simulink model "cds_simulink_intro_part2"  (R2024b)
settings: Solver=ode15s  StartTime=0.0  StopTime=30.0  RelTol=1e-3
undefined symbols (not defined in the file or in its folder): param

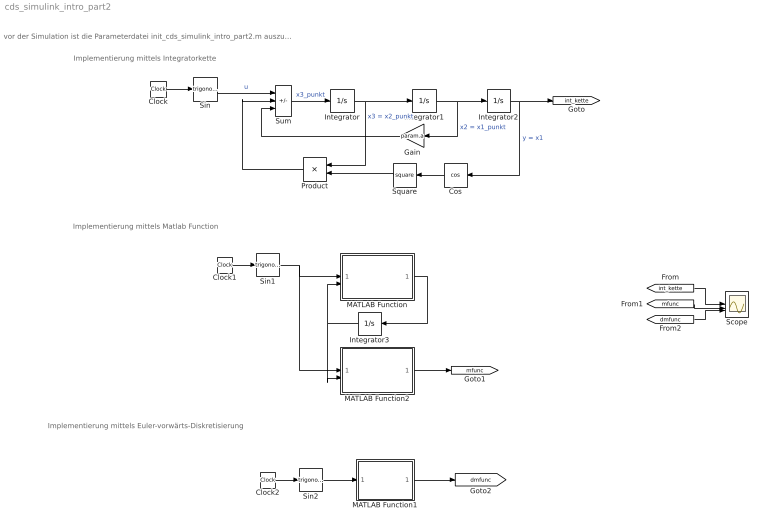
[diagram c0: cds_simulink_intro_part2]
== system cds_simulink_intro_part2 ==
  note: Implementierung mittels Matlab Function
  note: Implementierung mittels Integratorkette
  note: Implementierung mittels Euler-vorwärts-Diskretisierung
  note: vor der Simulation ist die Parameterdatei init_cds_simulink_intro_part2.m auszuführen
  Clock : Clock
  Clock1 : Clock
  Clock2 : Clock
  Cos : Trigonometry  Operator=cos
  Gain : Gain  Gain=param.a
  Integrator : Integrator
  Integrator1 : Integrator
  Integrator2 : Integrator
  Integrator3 : Integrator  InitialCondition=[0;0;0]
  MATLAB Function : MATLAB Function  TreatAsAtomicUnit=on
  MATLAB Function1 : MATLAB Function  TreatAsAtomicUnit=on
  MATLAB Function2 : MATLAB Function  TreatAsAtomicUnit=on
  Product : Product
  Scope : Scope  NumInputPorts=3
  Sin : Trigonometry
  Sin1 : Trigonometry
  Sin2 : Trigonometry
  Square : Math  Operator=square
  Sum : Sum  Inputs=---
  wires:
  Sin/1 -> Sum/1  "u"
  Integrator/1 -> Product/1, Integrator1/1  "x3 = x2_punkt"
  Sum/1 -> Integrator/1  "x3_punkt"
  Integrator1/1 -> Gain/1, Integrator2/1  "x2 = x1_punkt"
  Integrator2/1 -> [int_kette], Cos/1  "y = x1"
  Cos/1 -> Square/1
  Square/1 -> Product/2
  Product/1 -> Sum/2
  Clock/1 -> Sin/1
  Sin1/1 -> MATLAB Function2/1(u), MATLAB Function/1(u)
  Integrator3/1 -> MATLAB Function2/2(xx), MATLAB Function/2(xx)
  Clock1/1 -> Sin1/1
  Gain/1 -> Sum/3
  Clock2/1 -> Sin2/1
  Sin2/1 -> MATLAB Function1/1(u)
  MATLAB Function1/1(y) -> [dmfunc]
  [int_kette] -> Scope/1
  [mfunc] -> Scope/2
  [dmfunc] -> Scope/3
  MATLAB Function2/1(y) -> [mfunc]
  MATLAB Function/1(ff) -> Integrator3/1

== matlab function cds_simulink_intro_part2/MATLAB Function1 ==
function y = fcn(u,param)
   % Aufteilen der Parameter
   a = param.a;
   Ta = param.Ta;
	
   % Definition des diskreten Zustandes als persistent Variable
   persistent xx;
	
   % Initialisierung des diskreten Zustandes
   if isempty(xx); xx=param.xx0; end
	
   % Aufteilen des Zustandsvektors
   x1 = xx(1);
   x2 = xx(2);
   x3 = xx(3);
	
   % Implementierung von f(x,u)
   f1 = x2;
   f2 = x3;
   f3 = -cos(x1)^2*x3 -a*x2 -u;
	
   % Zusammenfuegen zu einem Vektor
   ff = [f1;
         f2;
         f3];

   % Approximation mittels Euler-Verfahren
   xx = xx + Ta*ff;
	
   % Implementierung von h(x,u)
   y = x1;
end

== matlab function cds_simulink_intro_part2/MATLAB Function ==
function ff  = Fcn(u,xx,param)
   % Aufteilen der Parameter (zur besseren Lesbarkeit)
   a = param.a;

   % Aufteilen des Zustandsvektors (zur besseren Lesbarkeit)
   x1 = xx(1);
   x2 = xx(2);
   x3 = xx(3);

   % Implementierung von f(x,u)
   f1 = x2;
   f2 = x3;
   f3 = -cos(x1)^2 * x3 - a*x2 -u;

   % Zuweisen des Ausgangs des Blocks f(x,u)
   ff = [f1;
         f2;
         f3];
end

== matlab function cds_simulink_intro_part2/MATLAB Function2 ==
function y  = fcn(u,xx,param)
	% Aufteilen der Parameter (zur besseren Lesbarkeit)
	a = param.a;
	
	% Aufteilen des Zustandsvektors (zur besseren Lesbarkeit)
	x1 = xx(1);
	x2 = xx(2);
	x3 = xx(3);

	% Implementierung von h(x,u)
	y = x1;
end
